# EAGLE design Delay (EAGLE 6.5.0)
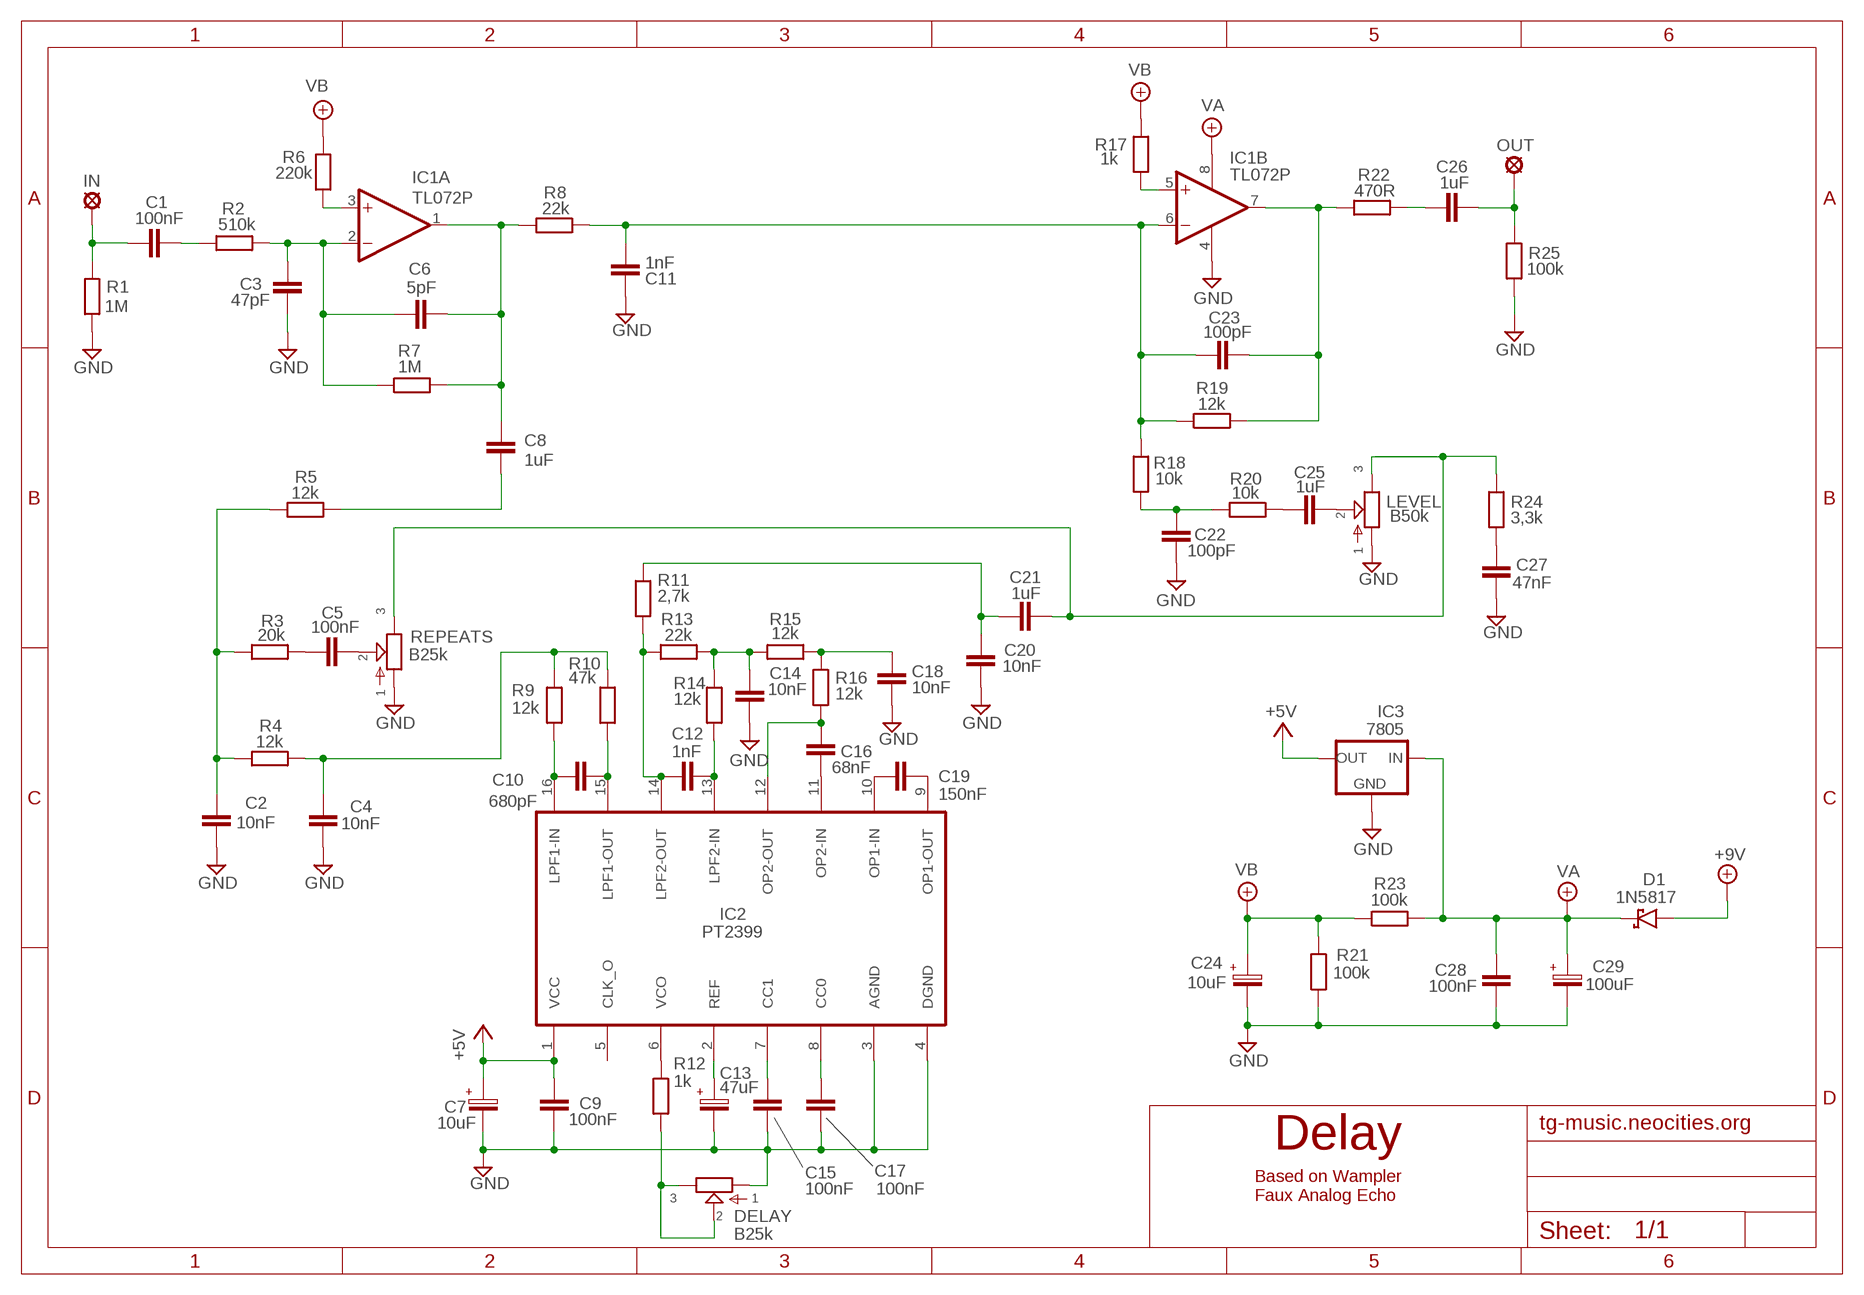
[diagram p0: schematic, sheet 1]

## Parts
+9V  +9V  +9V(T)1  [ROUND]
C1  100nF  072X0252  [072X025]
C2  10nF  072X0252  [072X025]
C3  47pF  050X030_0251  [050X030_025]
C4  10nF  072X0252  [072X025]
C5  100nF  072X0252  [072X025]
C6  5pF  050X030_0252  [050X030_025_2]
C7  10uF  050-EU1  [050_020_1]
C8  1uF  072X0352  [072X035]
C9  100nF  050X030_0251  [050X030_025]
C10  680pF  050X030_0252  [050X030_025_2]
C11  1nF  072X0252  [072X025]
C12  1nF  072X0252  [072X025]
C13  47uF  050-EU1  [050_020_1]
C14  10nF  072X0252  [072X025]
C15  100nF  050X030_0251  [050X030_025]
C16  68nF  072X0252  [072X025]
C17  100nF  050X030_0251  [050X030_025]
C18  10nF  072X0252  [072X025]
C19  150nF  072X0252  [072X025]
C20  10nF  072X0252  [072X025]
C21  1uF  072X0352  [072X035]
C22  100pF  050X030_0251  [050X030_025]
C23  100pF  050X030_0251  [050X030_025]
C24  10uF  050-EU1  [050_020_1]
C25  1uF  072X0352  [072X035]
C26  1uF  072X0352  [072X035]
C27  47nF  072X0252  [072X025]
C28  100nF  072X0252  [072X025]
C29  100uF  063-EU  [063_025]
D1  1N5817  [DO41-3]
DELAY  B25k  POT-EU16MM  [16MM]
GND  GND  GND(T)1  [ROUND]
IC1  TL072P  [DIL08]
IC2  PT2399  [DIL16]
IC3  7805  78LXX  [78LXX]
IN  MCS10B  [MCS10B]
LEVEL  B50k  POT-EU16MM  [16MM]
OUT  MCS10B  [MCS10B]
R1  1M  6MM-EU3  [R0207/3]
R2  510k  6MM-EU3  [R0207/3]
R3  20k  6MM-EU3  [R0207/3]
R4  12k  6MM-EU3  [R0207/3]
R5  12k  6MM-EU3  [R0207/3]
R6  220k  6MM-EU3  [R0207/3]
R7  1M  6MM-EU3  [R0207/3]
R8  22k  6MM-EU3  [R0207/3]
R9  12k  6MM-EU3  [R0207/3]
R10  47k  6MM-EU3  [R0207/3]
R11  2,7k  6MM-EU3  [R0207/3]
R12  1k  6MM-EU3  [R0207/3]
R13  22k  6MM-EU3  [R0207/3]
R14  12k  6MM-EU3  [R0207/3]
R15  12k  6MM-EU3  [R0207/3]
R16  12k  6MM-EU3  [R0207/3]
R17  1k  6MM-EU3  [R0207/3]
R18  10k  6MM-EU3  [R0207/3]
R19  12k  6MM-EU3  [R0207/3]
R20  10k  6MM-EU3  [R0207/3]
R21  100k  6MM-EU3  [R0207/3]
R22  470R  6MM-EU3  [R0207/3]
R23  100k  6MM-EU3  [R0207/3]
R24  3,3k  6MM-EU3  [R0207/3]
R25  100k  6MM-EU3  [R0207/3]
REPEATS  B25k  POT-EU16MM  [16MM]

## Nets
+5V: C7.+ C9.2 IC2.1(VCC) IC3.OUT
+9V: +9V.1(+9V) D1.A
GND: C2.1 C3.1 C4.1 C7.- C9.1 C11.1 C13.- C14.2 C15.2 C17.2 C18.2 C20.2 C22.1 C24.- C27.2 C28.1 C29.- DELAY.1 GND.1(GND) IC1.4(P:V-) IC2.3(AGND) IC2.4(DGND) IC3.GND LEVEL.1 R1.1 R21.2 R25.1 REPEATS.1
N$1: C19.2 IC2.9(OP1-OUT)
N$2: C19.1 IC2.10(OP1-IN)
N$3: C12.1 IC2.14(LPF2-OUT) R11.1 R13.1
N$4: C12.2 IC2.13(LPF2-IN) R14.1
N$5: C10.1 IC2.16(LPF1-IN) R9.1
N$6: C10.2 IC2.15(LPF1-OUT) R10.1
N$7: C17.1 IC2.8(CC0)
N$8: C15.1 IC2.7(CC1)
N$9: C1.1 IN.MP R1.2
N$10: C16.2 IC2.11(OP2-IN)
N$11: C16.1 IC2.12(OP2-OUT) R16.1
N$12: IC2.6(VCO) R12.2
N$13: C20.1 C21.1 R11.2
N$14: C1.2 R2.1
N$15: C27.1 R24.1
N$16: C3.2 C6.1 IC1.2(A:-IN) R2.2 R7.1
N$17: C13.+ IC2.2(REF)
N$18: DELAY.2 DELAY.3 R12.1
N$19: C6.2 C8.1 IC1.1(A:OUT) R7.2 R8.1
N$20: IC1.3(A:+IN) R6.1
N$21: C11.2 C23.1 IC1.6(B:-IN) R8.2 R18.2 R19.1
N$22: C23.2 IC1.7(B:OUT) R19.2 R22.1
N$24: C26.1 R22.2
N$26: C26.2 OUT.MP R25.2
N$27: C8.2 R5.2
N$28: C2.2 R3.1 R4.1 R5.1
N$29: C5.1 R3.2
N$30: C5.2 REPEATS.2
N$31: C4.2 R4.2 R9.2 R10.2
N$32: C22.2 R18.1 R20.1
N$33: C25.1 R20.2
N$34: C25.2 LEVEL.2
N$35: IC1.5(B:+IN) R17.1
N$36: C21.2 LEVEL.3 R24.2 REPEATS.3
N$37: C18.1 R15.2 R16.2
N$38: C14.1 R13.2 R14.2 R15.1
VA: C28.2 C29.+ D1.C IC1.8(P:V+) IC3.IN R23.1
VB: C24.+ R6.2 R17.2 R21.1 R23.2
Unconnected: IC2.5(CLK_O)

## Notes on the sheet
- tg-music.neocities.org
- Based on Wampler
  Faux Analog Echo

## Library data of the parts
+9V = gm-supply:+9V(T): +9V Voltage Supply
C1 C2 C4 C5 C11 C12 C14 C16 C18-C20 C27 C28 = Wima MKS:072X025: 1000pF - 0.47uF
C3 C6 C9 C10 C15 C17 C22 C23 = Keraamiset kondensaattorit:050X030_025: 47 - 120pF
C7 C13 C24 = Elektrolyytit:050-EU
C8 C21 C25 C26 = Wima MKS:072X035: 0.15 - 1.0uF;
C29 = Elektrolyytit:063-EU
D1 = Diodit:1N5817
DELAY LEVEL REPEATS = gm-pots:POT-EU
GND = gm-supply:GND(T): Ground
IC1 = Operaatiovahvistimet:TL072: OP AMP
IC2 = princeton-tech:PT2399: Echo Processor IC
IC3 = v-reg:78LXX: VOLTAGE REGULATOR
IN OUT = Padit:MCS10B: SOLDER PAD
R1-R25 = Vastukset:6MM-EU: 6mm Resistors (European schematic symbol)

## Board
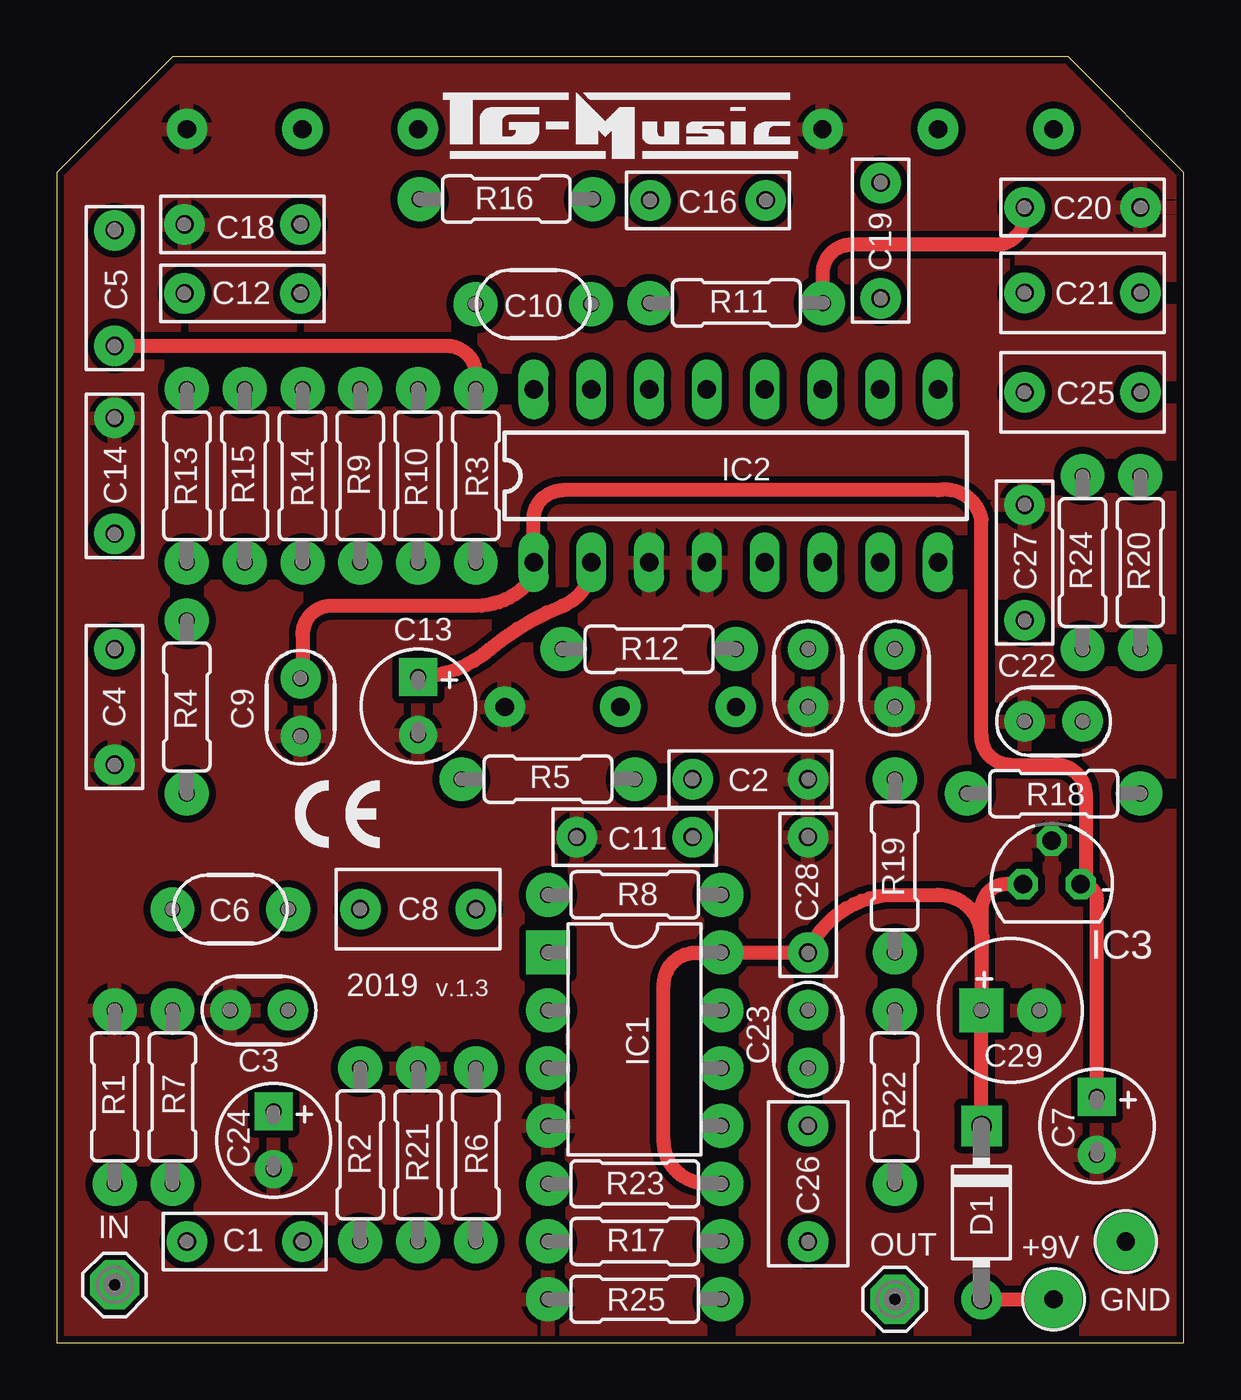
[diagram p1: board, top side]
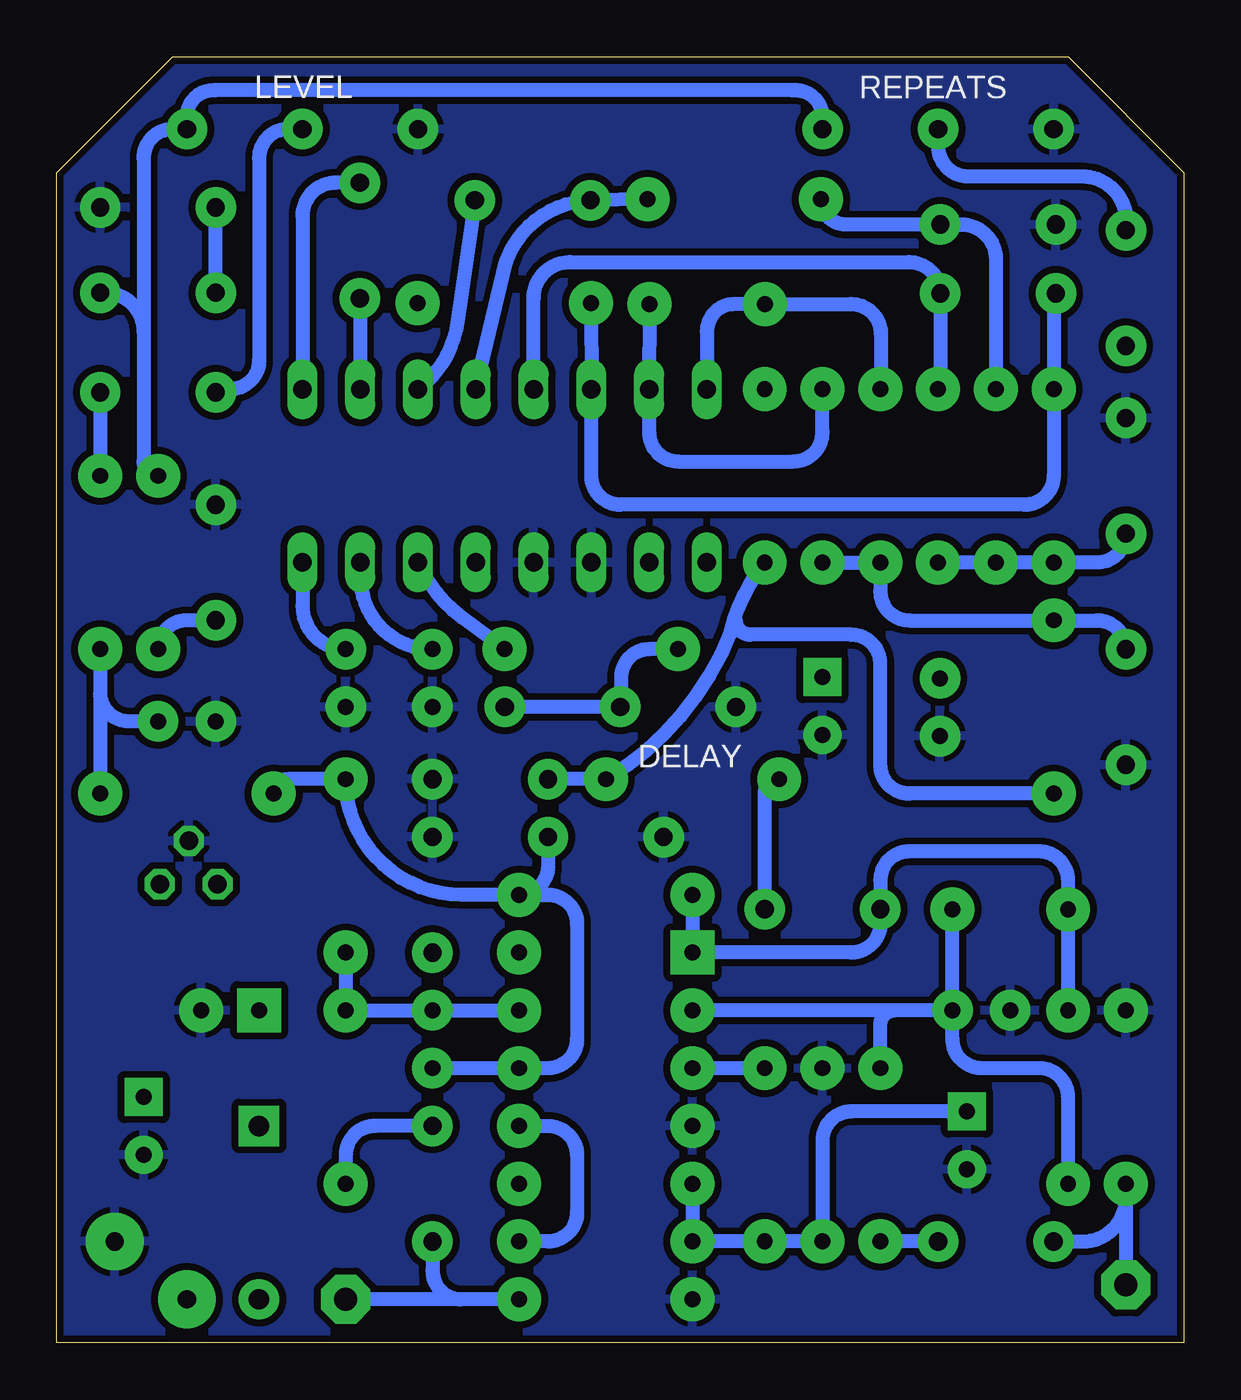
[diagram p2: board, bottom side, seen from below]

Size 49.53 x 56.52 mm. Coordinates in mm from the lower left corner, seen from the top.
Outline: 0,0 49.53,0 49.53,51.44 44.45,56.52 5.08,56.52 0,51.44 0,0
Copper layers (1*16): Top 0.035mm / dielectric 1.5mm / Bottom 0.035mm
Design rules "ITEADstudio": minimum track width 10mil, minimum drill 12mil, track to track 12mil, track to pad 12mil, pad to pad 12mil, via to via 12mil, smd to smd 0mil, copper to edge 12mil, drill to drill 12mil, minimum pad ring 10mil, minimum via ring 6mil, stop-mask expansion 4mil, vias tented up to drill 100mil, thermal gap 10mil

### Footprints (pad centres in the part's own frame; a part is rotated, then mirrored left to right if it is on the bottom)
ROUND = drill 0.8 pad 2.54: 1 0,0
072X025 = drill 0.8 pad 1.778: 1 -2.54,0; 2 2.54,0
050X030_025 = drill 0.7 pad 1.778: 1 -1.27,0; 2 1.27,0
050X030_025_2 = drill 0.7 pad 1.93: 1 -2.54,0; 2 2.54,0
050_020_1 = drill 0.7 pad 1.676 square: + -1.27,0 | drill 0.7 pad 1.676: - 1.27,0
072X035 = drill 0.8 pad 1.778: 1 -2.54,0; 2 2.54,0
063_025 = drill 0.7 pad 1.93 square: + -1.27,0 | drill 0.7 pad 1.93: - 1.27,0
DO41-3 = drill 0.9 pad 1.778: A 3.81,0 | drill 0.9 pad 1.778 square: C -3.81,0
16MM = drill 0.8 pad 1.778: 1 5.08,0; 2 0,0; 3 -5.08,0
DIL08 = drill 0.7 pad 1.93 square: 1 -3.81,-3.81 | drill 0.7 pad 1.93: 2 -1.27,-3.81; 3 1.27,-3.81; 4 3.81,-3.81; 5 3.81,3.81; 6 1.27,3.81; 7 -1.27,3.81; 8 -3.81,3.81
DIL16 = drill 0.813 long: 1 -8.89,-3.81; 2 -6.35,-3.81; 3 -3.81,-3.81; 4 -1.27,-3.81; 5 1.27,-3.81; 6 3.81,-3.81; 7 6.35,-3.81; 8 8.89,-3.81; 9 8.89,3.81; 10 6.35,3.81; 11 3.81,3.81; 12 1.27,3.81; 13 -1.27,3.81; 14 -3.81,3.81; 15 -6.35,3.81; 16 -8.89,3.81
78LXX = drill 0.813 octagon: GND 0,1.905; IN -1.27,0; OUT 1.27,0
MCS10B = drill 1.016 pad 2.159 octagon: MP 0,0
R0207/3 = drill 0.7 pad 1.93: 1 -3.81,0; 2 3.81,0

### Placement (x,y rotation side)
+9V  43.81,1.91 0 top
C1  8.26,4.45 0 top
C2  30.48,24.77 180 top
C3  8.89,14.61 0 top
C4  2.54,27.94 90 top
C5  2.54,46.35 90 top
C6  7.62,19.05 180 top
C7  45.72,9.53 270 top
C8  15.88,19.05 0 top
C9  10.71,27.93 90 top
C10  20.94,45.65 0 top
C11  25.4,22.23 0 top
C12  8.16,46.12 0 top
C13  15.88,27.98 270 top
C14  2.54,38.1 90 top
C15  33.02,29.21 270 top
C16  28.62,50.21 0 top
C17  36.83,29.21 270 top
C18  8.16,49.15 180 top
C19  36.21,48.44 90 top
C20  45.09,49.9 0 top
C21  45.09,46.15 0 top
C22  43.81,27.3 0 top
C23  33.02,13.34 90 top
C24  9.53,8.89 270 top
C25  45.09,41.77 180 top
C26  33.02,6.99 270 top
C27  42.55,34.29 90 top
C28  33.02,19.68 270 top
C29  41.91,14.61 0 top
D1  40.64,5.71 270 top
DELAY  24.77,27.94 180 top
GND  46.99,4.45 0 top
IC1  25.4,13.34 270 top
IC2  29.84,38.1 0 top
IC3  43.73,20.15 0 top
IN  2.54,2.54 0 top
LEVEL  38.73,53.34 180 top
OUT  36.83,1.91 0 top
R1  2.54,10.79 270 top
R2  13.34,8.26 90 top
R3  18.41,38.1 90 top
R4  5.71,27.94 90 top
R5  21.59,24.77 180 top
R6  18.41,8.26 270 top
R7  5.08,10.79 90 top
R8  25.4,19.68 0 top
R9  13.34,38.1 270 top
R10  15.88,38.1 270 top
R11  29.87,45.7 0 top
R12  26.04,30.48 0 top
R13  5.71,38.1 270 top
R14  10.79,38.1 270 top
R15  8.26,38.1 90 top
R16  19.75,50.27 180 top
R17  25.4,4.45 180 top
R18  43.81,24.13 180 top
R19  36.83,20.95 270 top
R20  47.62,34.29 90 top
R21  15.88,8.26 90 top
R22  36.83,10.79 270 top
R23  25.4,6.99 180 top
R24  45.09,34.29 90 top
R25  25.4,1.91 0 top
REPEATS  10.79,53.34 180 top

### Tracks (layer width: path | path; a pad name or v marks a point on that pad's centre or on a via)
+5V
  Top 0.61: C9.2 arc90 10.79,29.28 10.79,31.11 arc-90 12.06,32.38 18.41,32.38 arc37 20.32,33.02 arc53 IC2.1 20.95,36.2 arc-90 22.23,37.47 38.73,37.47 arc-90 40.64,36.2 40.64,26.67 arc90 41.91,25.4 43.9,25.4 arc-90 45.22,24.08 45.22,20.37 IC3.OUT arc-90 45.72,19.43 C7.+
+9V
  Top 0.61: D1.A +9V.1
GND
  pour Top: 0,0 0,51.44 5.08,56.52 44.45,56.52 49.53,51.44 49.53,0
  pour Bottom: 0,0 0,50.8 0,51.44 5.08,56.52 44.45,56.52 49.53,51.44 49.53,0
N$1
  Bottom 0.61: C19.2 37.28,50.98 arc-90 38.73,49.53 IC2.9
N$2
  Bottom 0.61: C19.1 IC2.10
N$3
  Bottom 0.61: R11.1 IC2.14 26.04,38.1 arc-90 24.77,36.83 6.99,36.83 arc-90 5.71,38.1 R13.1 5.71,46.02 arc90 C12.1
N$4
  Bottom 0.61: R14.1 arc-90 10.7,42.01 C12.2 arc-90 12.07,47.5 26.99,47.5 arc-90 28.57,45.91 IC2.13
N$5
  Bottom 0.61: R9.1 arc-90 13.31,41.93 13.31,44.35 arc-90 14.61,45.65 C10.1 19.75,45.65 arc-90 20.95,44.45 IC2.16
N$6
  Bottom 0.61: C10.2 IC2.15 23.5,40.01 arc-90 22.23,38.73 17.14,38.73 arc-90 15.88,40.01 R10.1
N$7
  Bottom 0.61: IC2.8 38.73,32.38 arc-90 C17.1
N$8
  Bottom 0.61: IC2.7 36.2,33.66 arc-90 C15.1
N$9
  Bottom 0.61: R1.2 2.54,6.35 | 2.54,6.35 2.54,3.17 arc90 IN.MP | C1.1 4.45,4.45 arc-90 2.54,6.35
N$10
  Bottom 0.61: C16.2 31.91,44.92 arc46 IC2.11
N$11
  Bottom 0.61: IC2.12 29.78,47.51 arc69 C16.1 R16.1
N$12
  Bottom 0.61: R12.2 31.71,31.87 arc29 IC2.6
N$13
  Top 0.61: R11.2 arc-90 33.66,45.72 33.66,46.99 arc-90 34.92,48.26 41.27,48.26 arc90 42.55,49.53 C20.1
  Bottom 0.61: C21.1 C20.1
N$14
  Bottom 0.61: C1.2 R2.1
N$15
  Bottom 0.61: C27.1 43.81,31.75 arc-90 R24.1
N$16
  Bottom 0.61: C3.2 C6.1 | R7.1 5.08,10.79 arc-90 6.35,12.06 8.89,12.06 arc90 10.16,13.34 C3.2 | C3.2 12.7,14.61 | 12.7,14.61 IC1.2 | R2.2 13.34,13.97 arc90 12.7,14.61
N$17
  Top 0.61: C13.+ arc39 19.05,30.48 arc-19 22.23,32.38 arc70 IC2.2
N$18
  Bottom 0.61: DELAY.3 DELAY.2 arc-90 24.73,27.98 24.73,29.24 arc90 23.49,30.48 R12.1
N$19
  Bottom 0.61: R8.1 IC1.1 14.61,17.14 arc-90 13.34,18.41 C8.1 13.34,20.32 arc90 12.06,21.59 6.35,21.59 arc90 5.08,20.32 C6.2 R7.2
N$20
  Bottom 0.61: R6.1 IC1.3
N$21
  Bottom 0.61: C23.1 IC1.6 27.94,12.06 arc-90 26.67,13.34 26.67,18.41 arc-90 27.94,19.68 R8.2 | C11.2 27.94,20.95 arc90 R8.2 | R18.2 arc90 39.37,24.77 R19.1 arc-90 31.75,19.68 R8.2
N$22
  Bottom 0.61: IC1.7 C23.2 R22.1 R19.2
N$24
  Bottom 0.61: C26.1 35.56,9.53 arc-90 36.83,8.26 R22.2
N$26
  Bottom 0.61: R25.2 31.75,1.91 | 31.75,1.91 OUT.MP | C26.2 33.02,3.17 arc-90 31.75,1.91
N$27
  Bottom 0.61: C8.2 18.41,24.13 arc90 R5.2
N$28
  Bottom 0.61: C2.2 R5.1 arc-38 19.92,31.23 | 19.92,31.23 arc24 R3.1 | R4.1 12.06,24.13 arc90 13.34,25.4 13.34,29.84 arc-90 14.61,31.11 19.05,31.11 arc90 19.68,31.75 19.68,31.46 arc90 19.92,31.23
N$29
  Top 0.61: C5.1 17.14,43.81 arc-90 18.41,42.55 R3.2
N$30
  Bottom 0.61: REPEATS.2 10.79,52.7 arc-90 9.56,51.26 4.48,51.26 arc90 2.54,49.36 C5.2
N$31
  Bottom 0.61: R10.2 R9.2 13.34,33.02 arc-90 12.06,31.75 R4.2 3.81,31.75 arc90 C4.2
N$32
  Bottom 0.61: R20.1 47.62,28.57 | 47.62,28.57 R18.1 | C22.2 46.35,27.3 arc90 47.62,28.57
N$33
  Bottom 0.61: C25.1 R20.2
N$34
  Bottom 0.61: LEVEL.2 39.37,53.34 arc-90 40.64,52.07 40.64,43.18 arc90 41.91,41.91 42.41,41.91 arc-90 C25.2
N$35
  Bottom 0.61: IC1.5 27.94,9.53 arc90 26.67,8.26 26.67,5.71 arc90 27.94,4.45 R17.1
N$36
  Bottom 0.61: REPEATS.3 15.88,53.98 arc-90 17.18,55.04 42.58,55.04 arc-90 43.81,53.98 LEVEL.3 44.45,53.34 arc-90 45.72,52.07 45.72,44.45 | 45.72,44.45 45.72,38.73 arc-90 R24.2 | C21.2 47.42,46.15 arc90 45.72,44.45
N$37
  Bottom 0.61: R15.2 8.26,47.62 arc-90 9.78,49.15 C18.1 14.86,49.15 arc92 R16.2
N$38
  Bottom 0.61: C14.1 arc90 3.81,34.29 R13.2 R15.1 R14.2
VA
  Top 0.61: D1.C C29.+ 40.64,17.78 | R23.1 28.57,6.99 arc-90 26.67,8.89 26.67,15.71 arc-90 28.1,17.14 29.14,17.14 arc90 29.14,17.14 IC1.8 C28.2 arc-67 36.83,19.68 38.73,19.68 arc-90 40.64,17.78 | 40.7,17.84 arc-90 40.64,17.78 | 40.69,17.85 arc90 40.7,17.84 | IC3.IN 41.74,20.15 arc90 40.64,19.05 40.64,17.9 arc90 40.7,17.84
VB
  Bottom 0.61: R23.2 R17.2 R6.2 R21.1 15.88,8.89 arc90 14.61,10.16 C24.+

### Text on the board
tNames: 2019 | v.1.3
